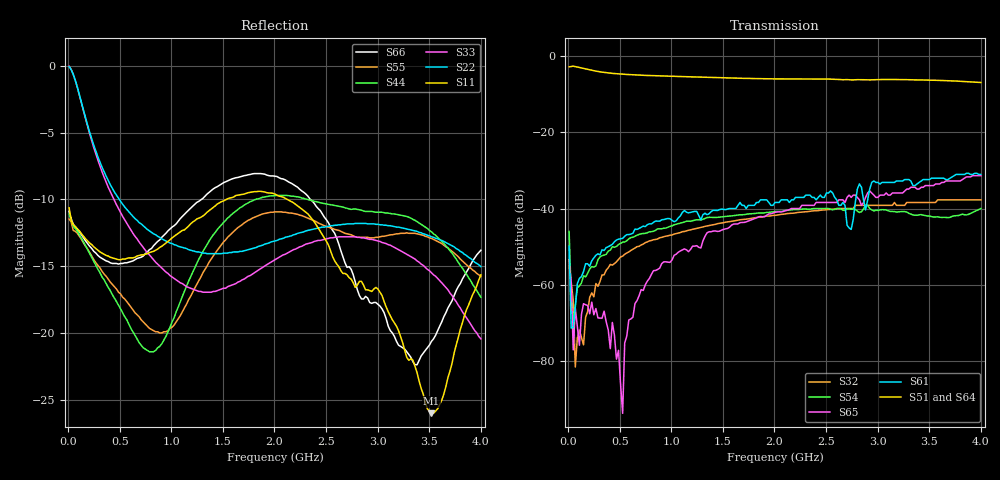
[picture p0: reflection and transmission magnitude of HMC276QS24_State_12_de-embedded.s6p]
! Hittite Microwave Corporation
! 20 Alpha Road
! Chelmsford, MA 01824
! Tel: 978-250-3343
! Fax: 978-250-3373
! Device: HMC276QS24, 0.7-3.0 GHz, GaAS MMIC 4x2 Switch Matrix in 24-lead QSOP package
! Misc: Data was de-embedded to package pins.
!  Port 1 = OP1
!  Port 2 = VL
!  Port 3 = VH
!  Port 4 = HH
!  Port 5 = HL
!  Port 6 = OP2
!  Vdd = +5 V
!  Vctl = 0 V[Logic 0] / +5 V[Logic 1]
!  State 12,  HL to OP1,  HH to OP2
!  Control Lines (Logic)
!  HV 1 = 1, Tone 1 = 0
!  HV 2 = 1, Tone 2 = 1
!  Data reformated to new Touchstone file format - Wed Jan 10 15:55:32 2007
# MHz S DB R 50
! 6 Port Network Data
! freq  dbS11  angS11  dbS12  angS12  dbS13  angS13  dbS14  angS14
!  dbS15  angS15  dbS16  angS16
!  dbS21  angS21  dbS22  angS22
!  dbS23  angS23  dbS24  angS24  dbS25  angS25  dbS26  angS26
!  dbS31  angS31  dbS32  angS32  dbS33  angS33  dbS34  angS34
!  dbS35  angS35  dbS36  angS36
!  dbS41  angS41  dbS42  angS42
!  dbS43  angS43  dbS44  angS44  dbS45  angS45  dbS46  angS46
!  dbS51  angS51  dbS52  angS52  dbS53  angS53  dbS54  angS54
!  dbS55  angS55  dbS56  angS56
!  dbS61  angS61  dbS62  angS62
!  dbS63  angS63  dbS64  angS64  dbS65  angS65  dbS66  angS66
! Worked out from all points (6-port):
!   201 points, 10 MHz to 4 GHz, reference 50 ohm
!   strongest paths, dB at 10 MHz, 1.008 GHz, 2.005 GHz, 3.002 GHz, 4 GHz:
!     S51: -2.8, -5.3, -6.0, -6.1, -6.9
!     S64: -2.8, -5.4, -6.2, -6.3, -7.0
!     S61: -49.9, -43.1, -38.4, -33.2, -31.1
!     S65: -53.4, -53.5, -41.0, -37.1, -31.4
!     S54: -46.0, -44.5, -40.8, -40.5, -40.0
!     S32: -55.1, -46.9, -41.8, -39.2, -37.7
!   lowest |S11| = -26.0 dB at 3.521 GHz (marker M1), VSWR 1.11, Z = 50.9 + j4.97 ohm
!   |S11| at or under -10 dB: start of sweep to 1.534 GHz; 2.123 GHz to end of sweep
